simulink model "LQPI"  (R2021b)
settings: Solver=VariableStepAuto  StartTime=0.0  StopTime=timeWaypoints(end)-0.2  RelTol=1e-3
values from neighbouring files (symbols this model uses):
  a = 0.27    [CompareGazeboSimulink.m]    (also in RobotModel.m)
  b = 0.31    [CompareGazeboSimulink.m]    (also in RobotModel.m)
  Dflag = 1    [RobotModel.m]
  distAng = 0    [RobotModel.m]
  distVel = 0    [RobotModel.m]
  fro = 0.02    [CompareGazeboSimulink.m]    (also in RobotModel.m)
  fsl = 0.8    [CompareGazeboSimulink.m]    (also in RobotModel.m)
  fsly = 0.8    [CompareGazeboSimulink.m]    (also in RobotModel.m)
  I = (1/12)*m*((2*t)^2 + 0.12^2) + 1.5    (= 2.384)    [CompareGazeboSimulink.m]    (also in RobotModel.m = 0.866666666667)
  Iflag = 1    [RobotModel.m]
  K = 22    [RobotModel.m]
  ko = 0    [CompareGazeboSimulink.m]    (also in RobotModel.m = 0.25)
  kt = 0.58    [CompareGazeboSimulink.m]    (also in RobotModel.m)
  m = 51    [CompareGazeboSimulink.m]    (also in RobotModel.m = 50)
  mdy = 10    [CompareGazeboSimulink.m]    (also in RobotModel.m)
  mst = 10    [CompareGazeboSimulink.m]    (also in RobotModel.m)
  N = 0    [RobotModel.m]
  Qt = [20 0 0    [RobotModel.m]
  r = 0.19    [CompareGazeboSimulink.m]    (also in RobotModel.m)
  Rt = [0.2 0    [RobotModel.m]
  T_vel_variance = 0.0005    [RobotModel.m]
  Td = 0.0125    [RobotModel.m]
  Th0 = 0    [CompareGazeboSimulink.m]    (also in RobotModel.m = 0.9714)
  Th_vel0 = 0    [CompareGazeboSimulink.m]    (also in RobotModel.m)
  Ti = 0.1    [RobotModel.m]
  timeWaypoints = [0, 3, 7.5, 10.5, 13.5, 18, 20.5]    [RobotModel.m]
  Ts = 0.01    [CompareGazeboSimulink.m]    (also in RobotModel.m = 0.05)
  waypoints = [0 5; 4 9; 8 1; 12 5; 8 9; 4 1; 0 5]    [CubicSpline.m]    (also in RobotModel.m = [0 2.5; 2 4.5; 4 0.5; 6 2.5; 4 4.5; 2 0.5; 0 2.5])
  X0 = 0    [CompareGazeboSimulink.m]    (also in RobotModel.m)
  x_vel0 = 0    [CompareGazeboSimulink.m]    (also in RobotModel.m)
  x_vel_variance = 0.0005    [RobotModel.m]
  Y0 = 0    [CompareGazeboSimulink.m]    (also in RobotModel.m = 2.5)
libraries: mobileRoboticsLib x1

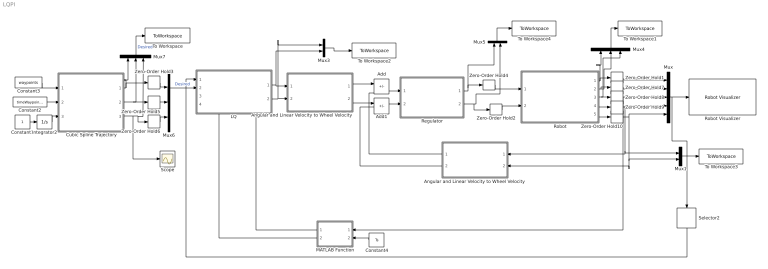
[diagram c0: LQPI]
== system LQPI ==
  Add : Sum  Inputs=+-
  Add1 : Sum  Inputs=+-
  Angular and Linear Velocity to Wheel Velocity : Subsystem
  "Angular and Linear Velocity to Wheel Velocity " : Subsystem
  Constant1 : Constant
  Constant2 : Constant  Value=timeWaypoints
  Constant3 : Constant  Value=waypoints
  Constant4 : Constant  Value=Ts
  Cubic Spline Trajectory : MATLAB Function  TreatAsAtomicUnit=on
  Integrator2 : Integrator
  "LQ " : Subsystem
  MATLAB Function : MATLAB Function  TreatAsAtomicUnit=on
  Mux : Mux  Inputs=5
  Mux1 : Mux  Inputs=2
  Mux3 : Mux  Inputs=2
  Mux4 : Mux  Inputs=3
  Mux5 : Mux  Inputs=2
  Mux6 : Mux  Inputs=3
  Mux7 : Mux  Inputs=3
  Regulator : Subsystem
  Robot : Subsystem
  Robot Visualizer : mobileRoboticsLib/Environments/Robot Visualizer  Commented=on  robotRadius=0.3  showTrajectory=on  hasWaypoints=off  hasLidar=off  sensorOffset=[ 0, 0 ]  scanAngles=[ -pi/4, 0, pi/4 ]  hasObjDetector=off  objDetectorOffset=[ 0, 0 ]  objDetectorAngle=0  objDetectorFOV=pi/4  objDetectorMaxRange=5  objectColors=[ 1, 0, 0; 0, 1, 0; 0, 0, 1 ]  objectMarkers=s
  Scope : Scope
  Selector2 : Selector  InputPortWidth=5  IndexOptions=Index vector (dialog)  Indices=[1 2 3]  OutputSizes=1
  To Workspace : ToWorkspace  VariableName=desiredPos  SaveFormat=Timeseries  SampleTime=-1
  To Workspace1 : ToWorkspace  VariableName=ActualPos  SaveFormat=Timeseries  SampleTime=-1
  To Workspace2 : ToWorkspace  VariableName=DesiredVel  SaveFormat=Timeseries  SampleTime=-1
  To Workspace3 : ToWorkspace  VariableName=ActualVel  SaveFormat=Timeseries  SampleTime=-1
  To Workspace4 : ToWorkspace  VariableName=Forces  SaveFormat=Timeseries  SampleTime=-1
  Zero-Order Hold{1..10} (10 alike) : ZeroOrderHold  SampleTime=Ts
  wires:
  Zero-Order Hold8/1 -> MATLAB Function/1(Theta), Mux/3
  Zero-Order Hold9/1 -> Mux1/1, "Angular and Linear Velocity to Wheel Velocity "/1(Angular Velocity), Mux/4
  Robot/3(Theta) -> Mux4/3, Zero-Order Hold8/1
  Mux1/1 -> To Workspace3/1
  Zero-Order Hold7/1 -> Mux/2
  Robot/4(Theta') -> Zero-Order Hold9/1
  Zero-Order Hold10/1 -> Mux1/2, "Angular and Linear Velocity to Wheel Velocity "/2(Linear Velocity), Mux/5
  Regulator/2(Right force action) -> Mux5/2, Zero-Order Hold2/1
  "Angular and Linear Velocity to Wheel Velocity "/1(wl) -> Add/2
  Robot/5(v) -> Zero-Order Hold10/1
  Mux5/1 -> To Workspace4/1
  Mux3/1 -> To Workspace2/1
  Zero-Order Hold1/1 -> Mux/1
  Robot/2(Y) -> Mux4/2, Zero-Order Hold7/1
  Mux4/1 -> To Workspace1/1
  Zero-Order Hold2/1 -> Robot/2(Right Force)
  Add1/1 -> Regulator/2(wr)
  Add/1 -> Regulator/1(wl)
  Angular and Linear Velocity to Wheel Velocity/1(wl) -> Add/1
  Robot/1(X) -> Mux4/1, Zero-Order Hold1/1
  Regulator/1(Left Force action) -> Mux5/1, Zero-Order Hold4/1
  Angular and Linear Velocity to Wheel Velocity/2("wr ") -> Add1/1
  Zero-Order Hold4/1 -> Robot/1(Left Force)
  "Angular and Linear Velocity to Wheel Velocity "/2("wr ") -> Add1/2
  Cubic Spline Trajectory/1(X) -> Mux7/1, Zero-Order Hold3/1
  Constant1/1 -> Integrator2/1
  Mux7/1 -> To Workspace/1  "Desired"
  Cubic Spline Trajectory/3(T) -> Scope/1, Mux7/3, Zero-Order Hold6/1
  Cubic Spline Trajectory/2(Y) -> Mux7/2, Zero-Order Hold5/1
  Zero-Order Hold5/1 -> Mux6/2
  Constant2/1 -> Cubic Spline Trajectory/2(time)
  Constant4/1 -> MATLAB Function/2(Ts)
  Constant3/1 -> Cubic Spline Trajectory/1(waypoints)
  MATLAB Function/1(A) -> "LQ "/4(A)
  Mux6/1 -> "LQ "/2(Desired State)  "Desired"
  Zero-Order Hold6/1 -> Mux6/3
  Integrator2/1 -> Cubic Spline Trajectory/3(actualTime)
  Zero-Order Hold3/1 -> Mux6/1
  MATLAB Function/2(B) -> "LQ "/3(B)
  Mux/1 -> Robot Visualizer/1, Selector2/1
  Selector2/1 -> "LQ "/1(Actual State)
  "LQ "/1(Linear Velocity) -> Mux3/2, Angular and Linear Velocity to Wheel Velocity/1(Linear Velocity)
  "LQ "/2("Angular Velocity ") -> Mux3/1, Angular and Linear Velocity to Wheel Velocity/2(Angular Velocity)

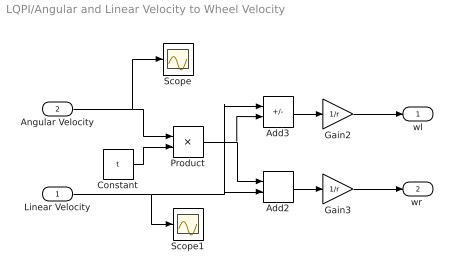
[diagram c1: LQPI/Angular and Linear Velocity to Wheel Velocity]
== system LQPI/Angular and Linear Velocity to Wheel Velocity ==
  Linear Velocity : Inport
  Angular Velocity : Inport  Port=2
  Add2 : Sum
  Add3 : Sum  Inputs=+-
  Constant : Constant  Value=t
  Gain2 : Gain  Gain=1/r
  Gain3 : Gain  Gain=1/r
  Product : Product
  Scope : Scope
  Scope1 : Scope
  wl : Outport
  "wr " : Outport  Port=2
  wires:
  Gain2/1 -> wl/1
  Linear Velocity/1 -> Scope1/1, Add2/2, Add3/1
  Gain3/1 -> "wr "/1
  Product/1 -> Add3/2, Add2/1
  Constant/1 -> Product/2
  Add3/1 -> Gain2/1
  Add2/1 -> Gain3/1
  Angular Velocity/1 -> Scope/1, Product/1

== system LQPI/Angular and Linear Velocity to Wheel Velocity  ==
  Angular Velocity : Inport
  Linear Velocity : Inport  Port=2
  Add2 : Sum
  Add3 : Sum  Inputs=+-
  Constant : Constant  Value=t
  Gain2 : Gain  Gain=1/r
  Gain3 : Gain  Gain=1/r
  Product : Product
  wl : Outport
  "wr " : Outport  Port=2
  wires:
  Angular Velocity/1 -> Product/1
  Add2/1 -> Gain3/1
  Add3/1 -> Gain2/1
  Constant/1 -> Product/2
  Product/1 -> Add2/1, Add3/2
  Gain3/1 -> "wr "/1
  Linear Velocity/1 -> Add3/1, Add2/2
  Gain2/1 -> wl/1

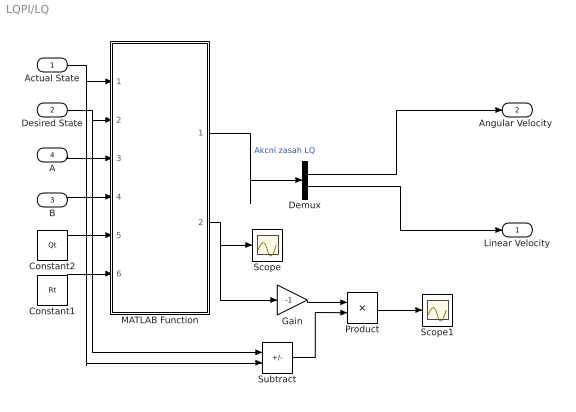
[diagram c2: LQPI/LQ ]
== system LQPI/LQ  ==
  Actual State : Inport
  Desired State : Inport  Port=2
  B : Inport  Port=3
  A : Inport  Port=4
  Constant1 : Constant  Value=Rt
  Constant2 : Constant  Value=Qt
  Demux : Demux  Outputs=2
  Gain : Gain  Gain=-1
  MATLAB Function : MATLAB Function  TreatAsAtomicUnit=on
  Product : Product  Multiplication=Matrix(*)
  Scope : Scope
  Scope1 : Scope
  Subtract : Sum  Inputs=+-
  Linear Velocity : Outport
  "Angular Velocity " : Outport  Port=2
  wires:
  Product/1 -> Scope1/1
  Gain/1 -> Product/1
  Subtract/1 -> Product/2
  Demux/2 -> Linear Velocity/1
  Demux/1 -> "Angular Velocity "/1
  MATLAB Function/2(K) -> Scope/1, Gain/1
  Constant1/1 -> MATLAB Function/6(R)
  Constant2/1 -> MATLAB Function/5(Q)
  B/1 -> MATLAB Function/4(B)
  A/1 -> MATLAB Function/3(A)
  Desired State/1 -> MATLAB Function/2(DesiredState), Subtract/1
  Actual State/1 -> MATLAB Function/1(ActualState), Subtract/2
  MATLAB Function/1(u) -> Demux/1  "Akcní zasah LQ"

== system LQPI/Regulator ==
  wl : Inport
  wr : Inport  Port=2
  PSDN : Subsystem
  PSDN1 : Subsystem
  Left Force action : Outport
  Right force action : Outport  Port=2
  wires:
  wl/1 -> PSDN/1(wl)
  PSDN/1(Left Force action) -> Left Force action/1
  wr/1 -> PSDN1/1(wr)
  PSDN1/1(Right force action) -> Right force action/1

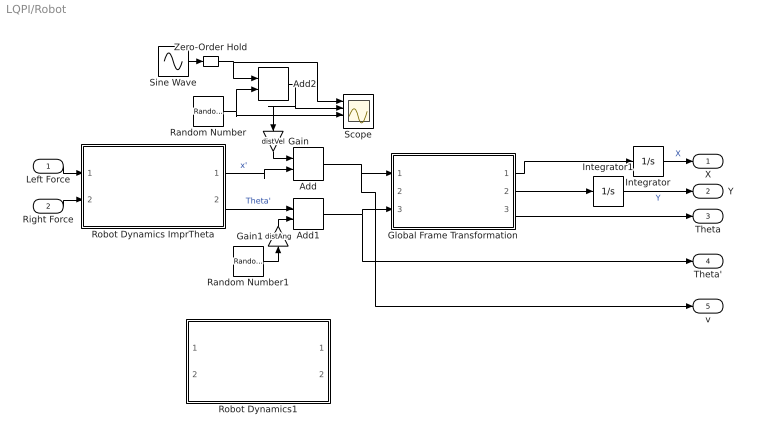
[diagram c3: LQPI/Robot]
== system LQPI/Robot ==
  Left Force : Inport
  Right Force : Inport  Port=2
  Add : Sum
  Add1 : Sum
  Add2 : Sum
  Gain : Gain  Gain=distVel
  Gain1 : Gain  Gain=distAng
  Global Frame Transformation : Subsystem
  Integrator : Integrator  InitialCondition=X0
  Integrator1 : Integrator  InitialCondition=Y0
  Random Number : RandomNumber  Variance=x_vel_variance  SampleTime=0.5
  Random Number1 : RandomNumber  Variance=T_vel_variance  SampleTime=0.1
  Robot Dynamics ImprTheta : Subsystem
  Robot Dynamics1 : Subsystem  Commented=on
  Scope : Scope  NumInputPorts=4
  Sine Wave : Sin  Amplitude=0.1  Frequency=0.2  SampleTime=0
  Zero-Order Hold : ZeroOrderHold  SampleTime=0.25
  X : Outport
  Y : Outport  Port=2
  Theta : Outport  Port=3
  Theta' : Outport  Port=4
  v : Outport  Port=5
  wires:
  Random Number/1 -> Add2/2, Scope/3
  Add2/1 -> Gain/1, Scope/2
  Gain/1 -> Add/1
  Sine Wave/1 -> Zero-Order Hold/1
  Add/1 -> v/1, Global Frame Transformation/1(x')
  Add1/1 -> Theta'/1, Global Frame Transformation/3(Theta')
  Random Number1/1 -> Gain1/1
  Left Force/1 -> Robot Dynamics ImprTheta/1(Left Force)
  Gain1/1 -> Add1/2
  Integrator1/1 -> Y/1  "Y"
  Zero-Order Hold/1 -> Scope/1, Add2/1
  Robot Dynamics ImprTheta/1(x') -> Add/2  "x'"
  Global Frame Transformation/2(Y') -> Integrator1/1
  Integrator/1 -> X/1  "X"
  Right Force/1 -> Robot Dynamics ImprTheta/2(Right Force)
  Global Frame Transformation/1(X') -> Integrator/1
  Global Frame Transformation/3(Theta) -> Theta/1
  Robot Dynamics ImprTheta/2(Theta') -> Add1/1  "Theta'"

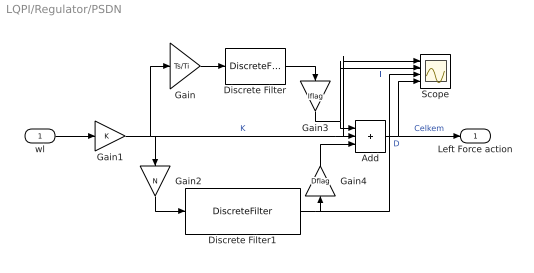
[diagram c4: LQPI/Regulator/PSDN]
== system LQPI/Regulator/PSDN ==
  wl : Inport
  Add : Sum  Inputs=3
  Discrete Filter : DiscreteFilter  Numerator=[0 1]  Denominator=[1 -1]
  Discrete Filter1 : DiscreteFilter  Numerator=[1 -1]  Denominator=[1 -exp(-Ts*N/Td)]
  Gain : Gain  Gain=Ts/Ti
  Gain1 : Gain  Gain=K
  Gain2 : Gain  Gain=N
  Gain3 : Gain  Gain=Iflag
  Gain4 : Gain  Gain=Dflag
  Scope : Scope  NumInputPorts=4
  Left Force action : Outport
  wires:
  Discrete Filter/1 -> Gain3/1
  Discrete Filter1/1 -> Scope/3, Gain4/1  "D"
  wl/1 -> Gain1/1
  Add/1 -> Left Force action/1, Scope/4  "Celkem"
  Gain/1 -> Discrete Filter/1
  Gain1/1 -> Gain2/1, Gain/1, Scope/1, Add/2  "K"
  Gain2/1 -> Discrete Filter1/1
  Gain3/1 -> Scope/2, Add/1  "I"
  Gain4/1 -> Add/3

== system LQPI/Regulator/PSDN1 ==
  wr : Inport
  Add : Sum  Inputs=3
  Discrete Filter : DiscreteFilter  Numerator=[0 1]  Denominator=[1 -1]
  Discrete Filter1 : DiscreteFilter  Numerator=[1 -1]  Denominator=[1 -exp(-Ts*N/Td)]
  Gain : Gain  Gain=Ts/Ti
  Gain1 : Gain  Gain=K
  Gain2 : Gain  Gain=N
  Gain3 : Gain  Gain=Iflag
  Gain4 : Gain  Gain=Dflag
  Right force action : Outport
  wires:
  Gain2/1 -> Discrete Filter1/1
  Gain1/1 -> Add/2, Gain/1, Gain2/1
  Gain/1 -> Discrete Filter/1
  Add/1 -> Right force action/1
  wr/1 -> Gain1/1
  Discrete Filter1/1 -> Gain4/1
  Discrete Filter/1 -> Gain3/1
  Gain3/1 -> Add/1
  Gain4/1 -> Add/3

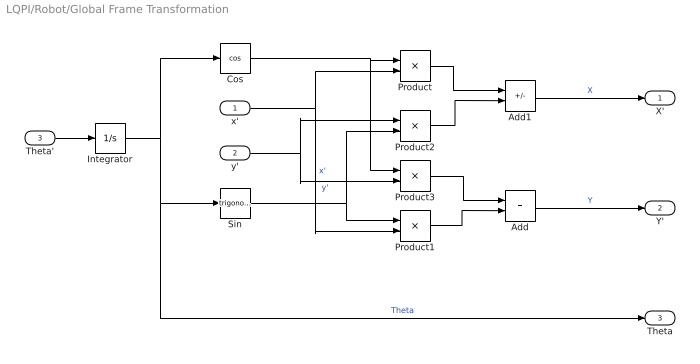
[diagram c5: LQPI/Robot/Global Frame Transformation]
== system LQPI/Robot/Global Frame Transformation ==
  x' : Inport
  y' : Inport  Port=2
  Theta' : Inport  Port=3
  Add : Sum
  Add1 : Sum  Inputs=+-
  Cos : Trigonometry  Operator=cos
  Integrator : Integrator  InitialCondition=Th0
  Product{,1..3} (4 alike) : Product
  Sin : Trigonometry
  X' : Outport
  Y' : Outport  Port=2
  Theta : Outport  Port=3
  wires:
  Add/1 -> Y'/1  "Y"
  Integrator/1 -> Theta/1, Sin/1, Cos/1  "Theta"
  Product1/1 -> Add/2
  x'/1 -> Product/2, Product1/2  "x'"
  Sin/1 -> Product1/1, Product2/2
  Product2/1 -> Add1/2
  Product3/1 -> Add/1
  Product/1 -> Add1/1
  Cos/1 -> Product/1, Product3/1
  y'/1 -> Product3/2, Product2/1  "y'"
  Add1/1 -> X'/1  "X"
  Theta'/1 -> Integrator/1

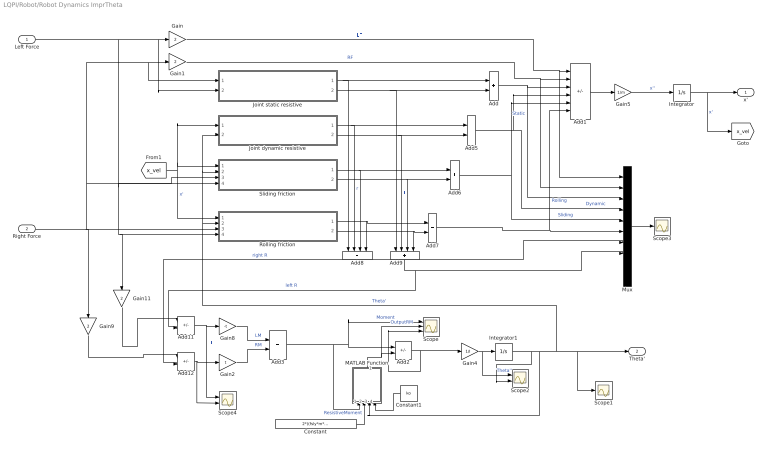
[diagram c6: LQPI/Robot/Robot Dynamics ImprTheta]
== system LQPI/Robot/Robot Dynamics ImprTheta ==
  Left Force : Inport
  Right Force : Inport  Port=2
  Add{,3,5..7} (5 alike) : Sum
  Add1 : Sum  Inputs=++----
  Add11 : Sum  Inputs=+-
  Add12 : Sum  Inputs=+-
  Add2 : Sum  Inputs=+-
  Add8 : Sum  Inputs=++++
  Add9 : Sum  Inputs=++++
  Constant : Constant  Value=2*((fsly*m*9.81)/(a+b))*a*b*kt
  Constant1 : Constant  Value=ko
  Gain{,1,9,11} (4 alike) : Gain  Gain=2
  Gain2 : Gain  Gain=t
  Gain4 : Gain  Gain=1/I
  Gain5 : Gain  Gain=1/m
  Gain8 : Gain  Gain=-t
  Integrator : Integrator  InitialCondition=x_vel0
  Integrator1 : Integrator  InitialCondition=Th_vel0
  Joint dynamic resistive : Subsystem
  Joint static resistive : Subsystem
  MATLAB Function : MATLAB Function  TreatAsAtomicUnit=on
  Mux : Mux  Inputs=10
  Rolling friction : Subsystem
  Scope : Scope  NumInputPorts=3
  Scope1 : Scope
  Scope2 : Scope  NumInputPorts=2
  Scope3 : Scope
  Scope4 : Scope  NumInputPorts=2
  Sliding friction : Subsystem
  x' : Outport
  Theta' : Outport  Port=2
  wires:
  Gain4/1 -> Scope2/1, Integrator1/1  "Theta''"
  Integrator1/1 -> Scope2/2, Sliding friction/2(Theta'), Joint dynamic resistive/2(Theta'), Rolling friction/2(Theta'), Scope1/1, Theta'/1, MATLAB Function/3(Omega)  "Theta'"
  Gain1/1 -> Mux/2, Add1/2  "RF"
  Add1/1 -> Gain5/1
  Gain5/1 -> Integrator/1  "x''"
  Integrator/1 -> x'/1, [x_vel]  "x'"
  [x_vel] -> Joint dynamic resistive/1("Local Long Velocity "), Sliding friction/1(Local longitudal velocity), Rolling friction/1(Local longitudal velocity)  "x'"
  Joint static resistive/2(Static Resistive Force Left) -> Add9/1, Add/2
  Joint dynamic resistive/1(Dynamic Resistive Force Right) -> Add8/2, Add5/1  "r"
  Joint dynamic resistive/2(Dynamic Resistive Force Left) -> Add9/2, Add5/2  "l"
  Sliding friction/1(Friction Right Force) -> Add8/3, Add6/1
  Sliding friction/2(Friction Left Force) -> Add9/3, Add6/2
  Rolling friction/1(Friction Right Force) -> Add8/4, Add7/1
  Rolling friction/2(Friction Left Force) -> Add9/4, Add7/2
  Add/1 -> Add1/3, Mux/3  "Static"
  Add6/1 -> Add1/5, Mux/5  "Sliding"
  Add7/1 -> Mux/6, Add1/6  "Rolling"
  Add5/1 -> Mux/4, Add1/4  "Dynamic"
  Add9/1 -> Add11/2, Mux/8  "left R"
  Add8/1 -> Add12/2, Mux/7  "right R"
  Mux/1 -> Scope3/1
  Add11/1 -> Scope4/1, Gain8/1  "LL"
  Add12/1 -> Scope4/2, Gain2/1
  Gain9/1 -> Add12/1
  Gain11/1 -> Add11/1
  Gain8/1 -> Add3/1  "LM"
  Gain2/1 -> Add3/2  "RM"
  Gain/1 -> Mux/1, Add1/1  "LF"
  Joint static resistive/1(Static Resistive Force Right) -> Add8/1, Add/1
  Add2/1 -> Scope/3, Gain4/1
  Add3/1 -> Scope/1, Add2/1, MATLAB Function/1(Moment)  "Moment"
  MATLAB Function/1(y) -> Scope/2, Add2/2  "OutputRM"
  Constant/1 -> MATLAB Function/2(ResistiveMoment)  "ResistiveMoment"
  Left Force/1 -> Gain11/1, Rolling friction/4(Fl), Sliding friction/4(Fl), Joint static resistive/2("Fl "), Gain/1
  Right Force/1 -> Gain9/1, Rolling friction/3(Fr), Sliding friction/3(Fr), Joint static resistive/1(Fr), Gain1/1
  Constant1/1 -> MATLAB Function/4(ko)

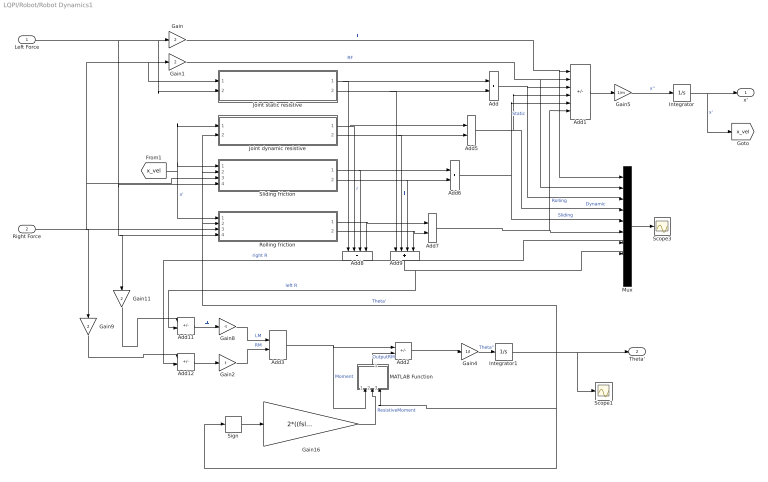
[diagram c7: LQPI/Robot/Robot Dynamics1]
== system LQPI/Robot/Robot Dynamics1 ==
  Left Force : Inport
  Right Force : Inport  Port=2
  Add{,3,5..7} (5 alike) : Sum
  Add1 : Sum  Inputs=++----
  Add11 : Sum  Inputs=+-
  Add12 : Sum  Inputs=+-
  Add2 : Sum  Inputs=+-
  Add8 : Sum  Inputs=++++
  Add9 : Sum  Inputs=++++
  Gain{,1,9,11} (4 alike) : Gain  Gain=2
  Gain16 : Gain  Gain=2*((fsly*m*9.81)/(a+b))*a*b
  Gain2 : Gain  Gain=t
  Gain4 : Gain  Gain=1/I
  Gain5 : Gain  Gain=1/m
  Gain8 : Gain  Gain=-t
  Integrator : Integrator  InitialCondition=x_vel0
  Integrator1 : Integrator  InitialCondition=Th_vel0
  Joint dynamic resistive : Subsystem
  Joint static resistive : Subsystem
  MATLAB Function : MATLAB Function  TreatAsAtomicUnit=on
  Mux : Mux  Inputs=10
  Rolling friction : Subsystem
  Scope1 : Scope
  Scope3 : Scope
  Sign : Signum
  Sliding friction : Subsystem
  x' : Outport
  Theta' : Outport  Port=2
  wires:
  Right Force/1 -> Rolling friction/3(Fr), Sliding friction/3(Fr), Joint static resistive/1(Fr), Gain1/1, Gain9/1
  Gain4/1 -> Integrator1/1  "Theta''"
  Integrator1/1 -> Sliding friction/2(Theta'), Joint dynamic resistive/2(Theta'), Rolling friction/2(Theta'), MATLAB Function/3(Omega), Sign/1, Scope1/1, Theta'/1  "Theta'"
  Left Force/1 -> Rolling friction/4(Fl), Gain11/1, Sliding friction/4(Fl), Joint static resistive/2("Fl "), Gain/1
  Gain1/1 -> Mux/2, Add1/2  "RF"
  Add1/1 -> Gain5/1
  Gain5/1 -> Integrator/1  "x''"
  Integrator/1 -> x'/1, [x_vel]  "x'"
  [x_vel] -> Joint dynamic resistive/1("Local Long Velocity "), Sliding friction/1(Local longitudal velocity), Rolling friction/1(Local longitudal velocity)  "x'"
  Joint static resistive/2(Static Resistive Force Left) -> Add9/1, Add/2
  Joint dynamic resistive/1(Dynamic Resistive Force Right) -> Add8/2, Add5/1  "r"
  Joint dynamic resistive/2(Dynamic Resistive Force Left) -> Add9/2, Add5/2  "l"
  Sliding friction/1(Friction Right Force) -> Add8/3, Add6/1
  Sliding friction/2(Friction Left Force) -> Add9/3, Add6/2
  Rolling friction/1(Friction Right Force) -> Add8/4, Add7/1
  Rolling friction/2(Friction Left Force) -> Add9/4, Add7/2
  Add/1 -> Add1/3, Mux/3  "Static"
  Add6/1 -> Add1/5, Mux/5  "Sliding"
  Add7/1 -> Mux/6, Add1/6  "Rolling"
  Add5/1 -> Mux/4, Add1/4  "Dynamic"
  Add9/1 -> Add11/2, Mux/8  "left R"
  Add8/1 -> Add12/2, Mux/7  "right R"
  Mux/1 -> Scope3/1
  Add11/1 -> Gain8/1  "LL"
  Add12/1 -> Gain2/1
  Gain9/1 -> Add12/1
  Gain11/1 -> Add11/1
  Gain8/1 -> Add3/1  "LM"
  Gain2/1 -> Add3/2  "RM"
  Gain/1 -> Mux/1, Add1/1  "LF"
  Joint static resistive/1(Static Resistive Force Right) -> Add8/1, Add/1
  Sign/1 -> Gain16/1
  Add2/1 -> Gain4/1
  Add3/1 -> Add2/1, MATLAB Function/1(Moment)  "Moment"
  MATLAB Function/1(y) -> Add2/2  "OutputRM"
  Gain16/1 -> MATLAB Function/2(ResistiveMoment)  "ResistiveMoment"

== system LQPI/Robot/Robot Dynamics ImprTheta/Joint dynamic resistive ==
  "Local Long Velocity " : Inport
  Theta' : Inport  Port=2
  Add2 : Sum  Inputs=+-
  Add5 : Sum
  Gain : Gain  Gain=(2*mdy)/(r*r)
  Gain1 : Gain  Gain=(2*mdy)/(r*r)
  Gain4 : Gain  Gain=t
  Scope : Scope  NumInputPorts=3
  Dynamic Resistive Force Right : Outport
  Dynamic Resistive Force Left : Outport  Port=2
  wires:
  Gain/1 -> Dynamic Resistive Force Right/1
  Gain1/1 -> Dynamic Resistive Force Left/1
  Gain4/1 -> Add5/2, Add2/2
  Theta'/1 -> Scope/3, Gain4/1
  Add5/1 -> Scope/2, Gain/1  "vr"
  Add2/1 -> Scope/1, Gain1/1  "vl"
  "Local Long Velocity "/1 -> Add2/1, Add5/1

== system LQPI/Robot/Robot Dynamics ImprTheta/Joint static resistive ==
  Fr : Inport
  "Fl " : Inport  Port=2
  Fsj : Gain  Gain=2*(mst/r)
  Fsj . : Gain  Gain=2*(mst/r)
  Gain1 : Gain  Gain=1/(mst/r)
  Gain2 : Gain  Gain=1/(mst/r)
  Tanh : Trigonometry  Operator=tanh
  Tanh1 : Trigonometry  Operator=tanh
  Static Resistive Force Right : Outport
  Static Resistive Force Left : Outport  Port=2
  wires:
  Fr/1 -> Gain1/1
  "Fl "/1 -> Gain2/1
  Tanh/1 -> Fsj/1
  Tanh1/1 -> Fsj ./1
  Gain1/1 -> Tanh/1
  Gain2/1 -> Tanh1/1
  Fsj/1 -> Static Resistive Force Right/1
  Fsj ./1 -> Static Resistive Force Left/1

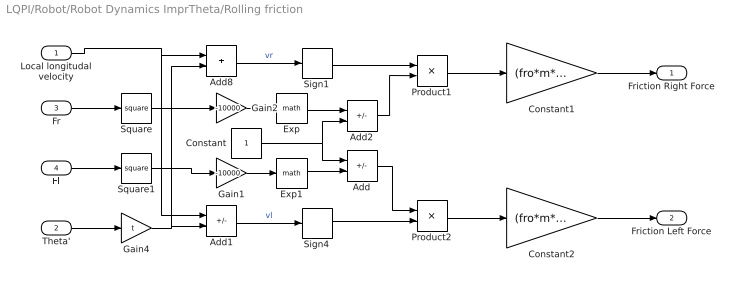
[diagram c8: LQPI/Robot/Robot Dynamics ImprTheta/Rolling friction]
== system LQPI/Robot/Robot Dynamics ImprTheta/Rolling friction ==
  Local longitudal velocity : Inport
  Theta' : Inport  Port=2
  Fr : Inport  Port=3
  Fl : Inport  Port=4
  Add : Sum  Inputs=+-
  Add1 : Sum  Inputs=+-
  Add2 : Sum  Inputs=-+
  Add8 : Sum
  Constant : Constant
  Constant1 : Gain  Gain=(fro*m*9.81)/2
  Constant2 : Gain  Gain=(fro*m*9.81)/2
  Exp : Math
  Exp1 : Math
  Gain1 : Gain  Gain=-10000
  Gain2 : Gain  Gain=-10000
  Gain4 : Gain  Gain=t
  Product1 : Product
  Product2 : Product
  Sign1 : Signum
  Sign4 : Signum
  Square : Math  Operator=square
  Square1 : Math  Operator=square
  Friction Right Force : Outport
  Friction Left Force : Outport  Port=2
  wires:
  Sign1/1 -> Product1/1
  Sign4/1 -> Product2/2
  Add8/1 -> Sign1/1  "vr"
  Fl/1 -> Square1/1
  Fr/1 -> Square/1
  Square1/1 -> Gain1/1
  Gain4/1 -> Add1/2, Add8/2
  Theta'/1 -> Gain4/1
  Add1/1 -> Sign4/1  "vl"
  Square/1 -> Gain2/1
  Gain2/1 -> Exp/1
  Gain1/1 -> Exp1/1
  Add2/1 -> Product1/2
  Add/1 -> Product2/1
  Exp1/1 -> Add/2
  Exp/1 -> Add2/1
  Constant/1 -> Add2/2, Add/1
  Local longitudal velocity/1 -> Add1/1, Add8/1
  Product1/1 -> Constant1/1
  Product2/1 -> Constant2/1
  Constant2/1 -> Friction Left Force/1
  Constant1/1 -> Friction Right Force/1

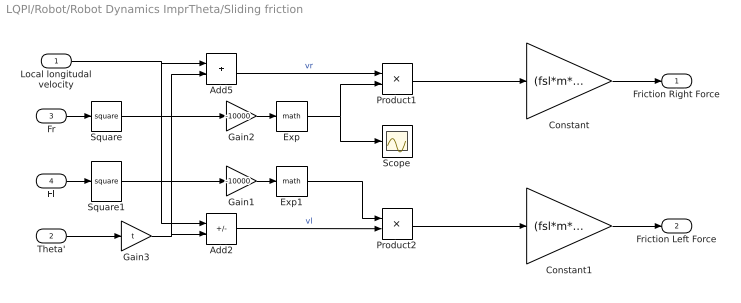
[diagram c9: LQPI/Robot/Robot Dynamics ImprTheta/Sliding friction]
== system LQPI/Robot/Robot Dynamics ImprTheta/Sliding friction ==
  Local longitudal velocity : Inport
  Theta' : Inport  Port=2
  Fr : Inport  Port=3
  Fl : Inport  Port=4
  Add2 : Sum  Inputs=+-
  Add5 : Sum
  Constant : Gain  Gain=(fsl*m*9.81)/2
  Constant1 : Gain  Gain=(fsl*m*9.81)/2
  Exp : Math
  Exp1 : Math
  Gain1 : Gain  Gain=-10000
  Gain2 : Gain  Gain=-10000
  Gain3 : Gain  Gain=t
  Product1 : Product
  Product2 : Product
  Scope : Scope
  Square : Math  Operator=square
  Square1 : Math  Operator=square
  Friction Right Force : Outport
  Friction Left Force : Outport  Port=2
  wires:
  Theta'/1 -> Gain3/1
  Gain3/1 -> Add2/2, Add5/2
  Add5/1 -> Product1/1  "vr"
  Add2/1 -> Product2/2  "vl"
  Exp/1 -> Scope/1, Product1/2
  Gain1/1 -> Exp1/1
  Gain2/1 -> Exp/1
  Fr/1 -> Square/1
  Fl/1 -> Square1/1
  Square/1 -> Gain2/1
  Square1/1 -> Gain1/1
  Product1/1 -> Constant/1
  Product2/1 -> Constant1/1
  Exp1/1 -> Product2/1
  Local longitudal velocity/1 -> Add2/1, Add5/1
  Constant/1 -> Friction Right Force/1
  Constant1/1 -> Friction Left Force/1

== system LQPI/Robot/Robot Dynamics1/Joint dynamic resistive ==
  "Local Long Velocity " : Inport
  Theta' : Inport  Port=2
  Add2 : Sum  Inputs=+-
  Add5 : Sum
  Gain : Gain  Gain=(2*mdy)/(r*r)
  Gain1 : Gain  Gain=(2*mdy)/(r*r)
  Gain4 : Gain  Gain=t
  Scope : Scope  NumInputPorts=3
  Dynamic Resistive Force Right : Outport
  Dynamic Resistive Force Left : Outport  Port=2
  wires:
  Gain/1 -> Dynamic Resistive Force Right/1
  Gain1/1 -> Dynamic Resistive Force Left/1
  Gain4/1 -> Add5/2, Add2/2
  Theta'/1 -> Scope/3, Gain4/1
  Add5/1 -> Scope/2, Gain/1  "vr"
  Add2/1 -> Scope/1, Gain1/1  "vl"
  "Local Long Velocity "/1 -> Add2/1, Add5/1

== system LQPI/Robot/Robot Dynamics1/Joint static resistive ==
  Fr : Inport
  "Fl " : Inport  Port=2
  Fsj : Gain  Gain=2*(mst/r)
  Fsj . : Gain  Gain=2*(mst/r)
  Gain1 : Gain  Gain=1/(mst/r)
  Gain2 : Gain  Gain=1/(mst/r)
  Tanh : Trigonometry  Operator=tanh
  Tanh1 : Trigonometry  Operator=tanh
  Static Resistive Force Right : Outport
  Static Resistive Force Left : Outport  Port=2
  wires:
  Fr/1 -> Gain1/1
  "Fl "/1 -> Gain2/1
  Tanh/1 -> Fsj/1
  Tanh1/1 -> Fsj ./1
  Gain1/1 -> Tanh/1
  Gain2/1 -> Tanh1/1
  Fsj/1 -> Static Resistive Force Right/1
  Fsj ./1 -> Static Resistive Force Left/1

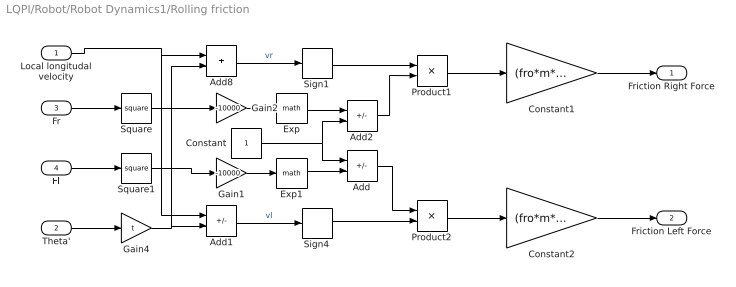
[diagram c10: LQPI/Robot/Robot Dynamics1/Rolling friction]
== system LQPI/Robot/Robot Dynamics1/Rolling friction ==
  Local longitudal velocity : Inport
  Theta' : Inport  Port=2
  Fr : Inport  Port=3
  Fl : Inport  Port=4
  Add : Sum  Inputs=+-
  Add1 : Sum  Inputs=+-
  Add2 : Sum  Inputs=-+
  Add8 : Sum
  Constant : Constant
  Constant1 : Gain  Gain=(fro*m*9.81)/2
  Constant2 : Gain  Gain=(fro*m*9.81)/2
  Exp : Math
  Exp1 : Math
  Gain1 : Gain  Gain=-10000
  Gain2 : Gain  Gain=-10000
  Gain4 : Gain  Gain=t
  Product1 : Product
  Product2 : Product
  Sign1 : Signum
  Sign4 : Signum
  Square : Math  Operator=square
  Square1 : Math  Operator=square
  Friction Right Force : Outport
  Friction Left Force : Outport  Port=2
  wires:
  Sign1/1 -> Product1/1
  Sign4/1 -> Product2/2
  Add8/1 -> Sign1/1  "vr"
  Fl/1 -> Square1/1
  Fr/1 -> Square/1
  Square1/1 -> Gain1/1
  Gain4/1 -> Add1/2, Add8/2
  Theta'/1 -> Gain4/1
  Add1/1 -> Sign4/1  "vl"
  Square/1 -> Gain2/1
  Gain2/1 -> Exp/1
  Gain1/1 -> Exp1/1
  Add2/1 -> Product1/2
  Add/1 -> Product2/1
  Exp1/1 -> Add/2
  Exp/1 -> Add2/1
  Constant/1 -> Add2/2, Add/1
  Local longitudal velocity/1 -> Add1/1, Add8/1
  Product1/1 -> Constant1/1
  Product2/1 -> Constant2/1
  Constant2/1 -> Friction Left Force/1
  Constant1/1 -> Friction Right Force/1

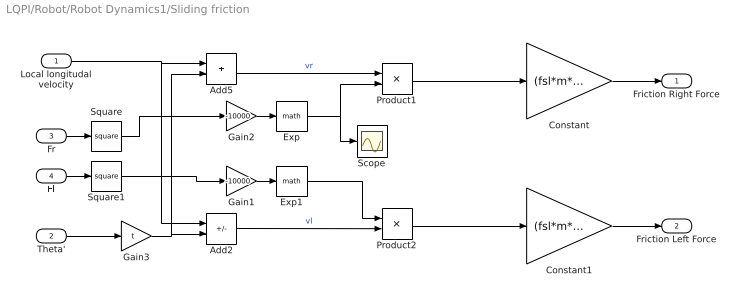
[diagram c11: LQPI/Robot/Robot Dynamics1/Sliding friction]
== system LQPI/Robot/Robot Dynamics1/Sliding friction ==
  Local longitudal velocity : Inport
  Theta' : Inport  Port=2
  Fr : Inport  Port=3
  Fl : Inport  Port=4
  Add2 : Sum  Inputs=+-
  Add5 : Sum
  Constant : Gain  Gain=(fsl*m*9.81)/2
  Constant1 : Gain  Gain=(fsl*m*9.81)/2
  Exp : Math
  Exp1 : Math
  Gain1 : Gain  Gain=-10000
  Gain2 : Gain  Gain=-10000
  Gain3 : Gain  Gain=t
  Product1 : Product
  Product2 : Product
  Scope : Scope
  Square : Math  Operator=square
  Square1 : Math  Operator=square
  Friction Right Force : Outport
  Friction Left Force : Outport  Port=2
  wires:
  Theta'/1 -> Gain3/1
  Gain3/1 -> Add2/2, Add5/2
  Add5/1 -> Product1/1  "vr"
  Add2/1 -> Product2/2  "vl"
  Exp/1 -> Scope/1, Product1/2
  Gain1/1 -> Exp1/1
  Gain2/1 -> Exp/1
  Fr/1 -> Square/1
  Fl/1 -> Square1/1
  Square/1 -> Gain2/1
  Square1/1 -> Gain1/1
  Product1/1 -> Constant/1
  Product2/1 -> Constant1/1
  Exp1/1 -> Product2/1
  Local longitudal velocity/1 -> Add2/1, Add5/1
  Constant/1 -> Friction Right Force/1
  Constant1/1 -> Friction Left Force/1

== matlab function LQPI/Cubic Spline
Trajectory ==
function [X, Y, T] = TrajectoryGeneration(waypoints, time, actualTime)
%% Cubic spline
t = time;
Ax = zeros((size(waypoints,1)-1)*4);
Bx = zeros((size(waypoints,1)-1)*4, 1);

Ay = zeros((size(waypoints,1)-1)*4);
By = zeros((size(waypoints,1)-1)*4, 1);

%% Start and End Points (1-10)
% First polynom
Ax(1,1:4) = [t(1)^3 t(1)^2 t(1) 1];
Ax(2,1:4) = [t(2)^3 t(2)^2 t(2) 1];
Bx(1) = waypoints(1,1);
Bx(2) = waypoints(2,1);

Ay(1,1:4) = [t(1)^3 t(1)^2 t(1) 1];
Ay(2,1:4) = [t(2)^3 t(2)^2 t(2) 1];
By(1) = waypoints(1,2);
By(2) = waypoints(2,2);

% Second polynom
Ax(3,5:8) = [t(2)^3 t(2)^2 t(2) 1];
Ax(4,5:8) = [t(3)^3 t(3)^2 t(3) 1];
Bx(3) = waypoints(2,1);
Bx(4) = waypoints(3,1);

Ay(3,5:8) = [t(2)^3 t(2)^2 t(2) 1];
Ay(4,5:8) = [t(3)^3 t(3)^2 t(3) 1];
By(3) = waypoints(2,2);
By(4) = waypoints(3,2);

% Third polynom
Ax(5,9:12) = [t(3)^3 t(3)^2 t(3) 1];
Ax(6,9:12) = [t(4)^3 t(4)^2 t(4) 1];
Bx(5) = waypoints(3,1);
Bx(6) = waypoints(4,1);

Ay(5,9:12) = [t(3)^3 t(3)^2 t(3) 1];
Ay(6,9:12) = [t(4)^3 t(4)^2 t(4) 1];
By(5) = waypoints(3,2);
By(6) = waypoints(4,2);

% Fourth polynom
Ax(7,13:16) = [t(4)^3 t(4)^2 t(4) 1];
Ax(8,13:16) = [t(5)^3 t(5)^2 t(5) 1];
Bx(7) = waypoints(4,1);
Bx(8) = waypoints(5,1);

Ay(7,13:16) = [t(4)^3 t(4)^2 t(4) 1];
Ay(8,13:16) = [t(5)^3 t(5)^2 t(5) 1];
By(7) = waypoints(4,2);
By(8) = waypoints(5,2);

% Fifth polynom
Ax(9,17:20) = [t(5)^3 t(5)^2 t(5) 1];
Ax(10,17:20) = [t(6)^3 t(6)^2 t(6) 1];
Bx(9) = waypoints(5,1);
Bx(10) = waypoints(6,1);

Ay(9,17:20) = [t(5)^3 t(5)^2 t(5) 1];
Ay(10,17:20) = [t(6)^3 t(6)^2 t(6) 1];
By(9) = waypoints(5,2);
By(10) = waypoints(6,2);

% Sixth polynom
Ax(11,21:24) = [t(6)^3 t(6)^2 t(6) 1];
Ax(12,21:24) = [t(7)^3 t(7)^2 t(7) 1];
Bx(11) = waypoints(6,1);
Bx(12) = waypoints(7,1);

Ay(11,21:24) = [t(6)^3 t(6)^2 t(6) 1];
Ay(12,21:24) = [t(7)^3 t(7)^2 t(7) 1];
By(11) = waypoints(6,2);
By(12) = waypoints(7,2);

%% First derivation (11-14)
Ax(13, 1:8) = [3*t(2)^2 2*t(2) 1 0 -3*t(2)^2 -2*t(2) -1 0];
Ax(14, 5:12) = [3*t(3)^2 2*t(3) 1 0 -3*t(3)^2 -2*t(3) -1 0];
Ax(15, 9:16) = [3*t(4)^2 2*t(4) 1 0 -3*t(4)^2 -2*t(4) -1 0];
Ax(16, 13:20) = [3*t(5)^2 2*t(5) 1 0 -3*t(5)^2 -2*t(5) -1 0];
Ax(17, 17:24) = [3*t(6)^2 2*t(6) 1 0 -3*t(6)^2 -2*t(6) -1 0];

Ay(13, 1:8) = [3*t(2)^2 2*t(2) 1 0 -3*t(2)^2 -2*t(2) -1 0];
Ay(14, 5:12) = [3*t(3)^2 2*t(3) 1 0 -3*t(3)^2 -2*t(3) -1 0];
Ay(15, 9:16) = [3*t(4)^2 2*t(4) 1 0 -3*t(4)^2 -2*t(4) -1 0];
Ay(16, 13:20) = [3*t(5)^2 2*t(5) 1 0 -3*t(5)^2 -2*t(5) -1 0];
Ay(17, 17:24) = [3*t(6)^2 2*t(6) 1 0 -3*t(6)^2 -2*t(6) -1 0];

%% Second derivation (15-18)
Ax(18, 1:8) = [6*t(2) 2 0 0 -6*t(2) -2 0 0];
Ax(19, 5:12) = [6*t(3) 2 0 0 -6*t(3) -2 0 0];
Ax(20, 9:16) = [6*t(4) 2 0 0 -6*t(4) -2 0 0];
Ax(21, 13:20) = [6*t(5) 2 0 0 -6*t(5) -2 0 0];
Ax(22, 17:24) = [6*t(6) 2 0 0 -6*t(6) -2 0 0];

Ay(18, 1:8) = [6*t(2) 2 0 0 -6*t(2) -2 0 0];
Ay(19, 5:12) = [6*t(3) 2 0 0 -6*t(3) -2 0 0];
Ay(20, 9:16) = [6*t(4) 2 0 0 -6*t(4) -2 0 0];
Ay(21, 13:20) = [6*t(5) 2 0 0 -6*t(5) -2 0 0];
Ay(22, 17:24) = [6*t(6) 2 0 0 -6*t(6) -2 0 0];

%% Initial condition (19-20)
Ax(23, 1:4) = [3*t(1)^2 2*t(1) 1 0];
Ax(24, 21:24) = [3*t(end)^2 2*t(end) 1 0];
Bx(23) = 0;
Bx(24) = 0;

Ay(23, 1:4) = [3*t(1)^2 2*t(1) 1 0];
Ay(24, 21:24) = [3*t(end)^2 2*t(end) 1 0];
By(23) = 0;
By(24) = 0;

%% Solve equation
Px = Ax \ Bx;
Py = Ay \ By;

if(actualTime <= t(2))
    X = [actualTime^3 actualTime^2 actualTime 1]*Px(1:4);
    Y = [actualTime^3 actualTime^2 actualTime 1]*Py(1:4);
    Xd = [3*actualTime^2 2*actualTime 1 0]*Px(1:4);
    Yd = [3*actualTime^2 2*actualTime 1 0]*Py(1:4);
elseif(actualTime <= t(3))
    X = [actualTime^3 actualTime^2 actualTime 1]*Px(5:8);
    Y = [actualTime^3 actualTime^2 actualTime 1]*Py(5:8);
    Xd = [3*actualTime^2 2*actualTime 1 0]*Px(5:8);
    Yd = [3*actualTime^2 2*actualTime 1 0]*Py(5:8);
elseif(actualTime <= t(4))
    X = [actualTime^3 actualTime^2 actualTime 1]*Px(9:12);
    Y = [actualTime^3 actualTime^2 actualTime 1]*Py(9:12);
    Xd = [3*actualTime^2 2*actualTime 1 0]*Px(9:12);
    Yd = [3*actualTime^2 2*actualTime 1 0]*Py(9:12);
elseif(actualTime <= t(5))
    X = [actualTime^3 actualTime^2 actualTime 1]*Px(13:16);
    Y = [actualTime^3 actualTime^2 actualTime 1]*Py(13:16);
    Xd = [3*actualTime^2 2*actualTime 1 0]*Px(13:16);
    Yd = [3*actualTime^2 2*actualTime 1 0]*Py(13:16);
elseif(actualTime <= t(6))
    X = [actualTime^3 actualTime^2 actualTime 1]*Px(17:20);
    Y = [actualTime^3 actualTime^2 actualTime 1]*Py(17:20);
    Xd = [3*actualTime^2 2*actualTime 1 0]*Px(17:20);
    Yd = [3*actualTime^2 2*actualTime 1 0]*Py(17:20);
else
    X = [actualTime^3 actualTime^2 actualTime 1]*Px(21:24);
    Y = [actualTime^3 actualTime^2 actualTime 1]*Py(21:24);
    Xd = [3*actualTime^2 2*actualTime 1 0]*Px(21:24);
    Yd = [3*actualTime^2 2*actualTime 1 0]*Py(21:24);
end    
    persistent Theta;
    persistent al;
    if isempty(al)
        al = 0.9714;
        Theta = al;
        a = al;
    else
        a = atan2(Yd, Xd);
    end
    if(al > 0 && a < 0 && al > pi/2)
        Theta = Theta + a - al + 2*pi;
    elseif(al < 0 && a > 0 && al < -pi/2)
        Theta = Theta + a - al - 2*pi;
    else
        Theta = Theta + a - al;
    end

    al = a;
    T = Theta;

end

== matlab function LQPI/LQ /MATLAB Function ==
function [u, K]   = lqTracking(ActualState, DesiredState, A, B, Q, R)                                                     

K_old = [ 0 0 0;
          0 0 0];
K     = [1 1 1;
         1 1 1];

% Co = ctrb(A,B); 
% unco = length(A) - rank(Co);

P = Q;
i = 0;
while (K ~= K_old)
    i = i + 1;
    K_old = K;
    P = Q + K'*R*K + (A - B*K)'*P*(A - B*K);
    K = (R + B'*P*B)^(-1)*B'*P*A;

    if (i > 100)
        break
    end
end

u = -K*(ActualState-DesiredState);
end

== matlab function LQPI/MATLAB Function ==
function [A, B] = fcn(Theta, Ts)
    
    A = eye(3);
    B = Ts*[0 cos(Theta); 0 sin(Theta); 1 0];
end

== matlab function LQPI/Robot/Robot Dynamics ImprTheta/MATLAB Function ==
function y = fcn(Moment, ResistiveMoment, Omega, ko)
    y = Omega*ResistiveMoment;

%     if(abs(Moment) < abs(ResistiveMoment))
%         y = Moment;
%     else
%         y = (ko*Omega + sign(Omega))*ResistiveMoment;
%     end



end

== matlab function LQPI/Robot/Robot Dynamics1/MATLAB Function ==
function y = fcn(Moment, ResistiveMoment, Omega)
    y = ResistiveMoment;
    
    if(Omega ~= 0)
        if(abs(Moment) < abs(ResistiveMoment))
            y = sign(Omega)*abs(Moment);
        else
            y = ResistiveMoment;
        end
    else
        y = 0;


end
